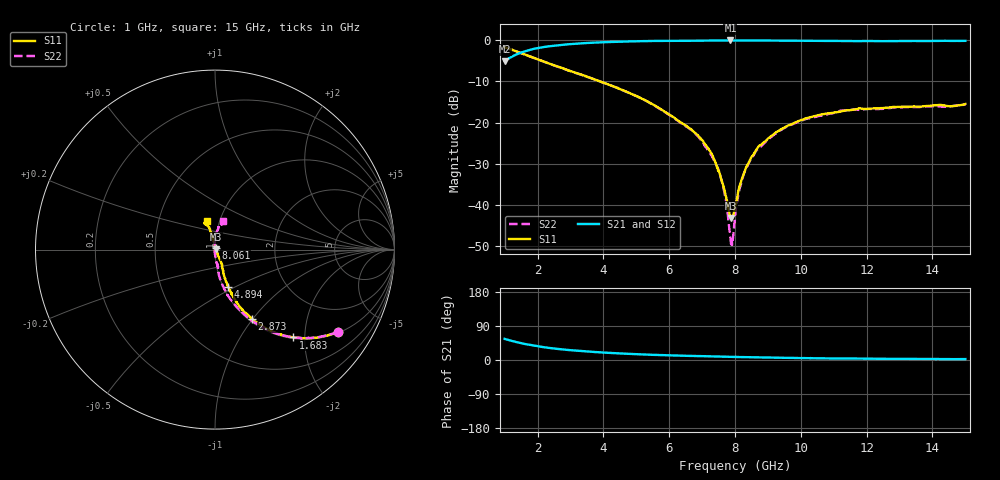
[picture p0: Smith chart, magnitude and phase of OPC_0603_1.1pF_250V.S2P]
! FILE NAME
! DATE 08/21/2012  11:30
! CORRECTED  DATA
# GHz  S  MA  R  50.00
!  FREQ  S11M  S11A  S21M  S21A  S12M  S12A  S22M  S22A
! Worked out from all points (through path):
!   1601 points, 1 GHz to 15 GHz, reference 50 ohm
!   highest |S21| = -0.06 dB at 7.86 GHz (marker M1); lowest = -5.1 dB at 1 GHz (marker M2)
!   group delay of S21, straight-line fit = 7.3 ps
!   lowest |S11| = -43.2 dB at 7.886 GHz (marker M3), VSWR 1.01, Z = 50.7 + j0.169 ohm
!   |S11| at or under -10 dB: 3.891 GHz to end of sweep
!   |S22| runs from -50.0 to -1.7 dB; largest |S21 - S12| = 0.0083
!   S11 on the Smith chart (normalised r, x): 1 GHz: 1.03, -2.96; 1.683 GHz: 1.02, -1.76; 2.873 GHz: 1.03, -0.99; 4.894 GHz: 1.06, -0.46; 8.061 GHz: 1.01, +0.02; 15 GHz: 0.87, +0.29
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1  0.8241 -33.9  0.5547 55.8  0.5546 55.7  0.8237 -33.8
1.6825  0.6553 -48.3  0.7453 41.3  0.7451 41.3  0.6545 -48.4
2.8725  0.4391 -62.0  0.8891 26.9  0.8891 26.9  0.4385 -63.2
3.33625  0.3806 -64.9  0.9159 23.6  0.9157 23.6  0.379 -66.8
4.89375  0.2198 -70.3  0.9678 15.8  0.9677 15.8  0.2187 -77.1
5.6725  0.1514 -70.8  0.9804 13.1  0.9803 13.1  0.1505 -81.0
6.73125  0.07781 -64.2  0.9837 10.7  0.9832 10.7  0.07707 -82.1
7.32625  0.03881 -63.5  0.991 9.5  0.9906 9.5  0.03683 -86.7
7.4925  0.02576 -57.9  0.9909 9.1  0.9906 9.1  0.02693 -90.1
7.64125  0.01723 -47.7  0.9916 8.8  0.9912 8.8  0.01676 -95.8
7.72875  0.01251 -37.0  0.9918 8.6  0.9917 8.6  0.0112 -100.4
7.86  0.00719 1.6  0.9926 8.4  0.9919 8.4  0.003987 -137.9
7.88625  0.006935 13.9  0.9922 8.3  0.9922 8.3  0.003253 -169.9
7.93875  0.007192 39.7  0.9921 8.2  0.992 8.2  0.003941 128.8
8  0.009706 61.5  0.9924 8.1  0.9915 8.1  0.007209 118.2
8.06125  0.01196 76.2  0.9923 8.0  0.9919 8.0  0.01094 107.7
8.30625  0.02624 93.8  0.9913 7.5  0.9911 7.5  0.02578 95.7
8.67375  0.04834 99.2  0.9904 7.0  0.9902 7.0  0.04661 89.9
9.4875  0.08638 102.3  0.9882 5.8  0.988 5.8  0.08533 86.2
10.33625  0.1173 104.0  0.9838 4.7  0.9833 4.7  0.1144 81.5
12.6725  0.1522 110.9  0.9724 3.3  0.9725 3.3  0.1494 76.7
15  0.1677 105.7  0.9818 2.5  0.9816 2.5  0.1658 74.8
